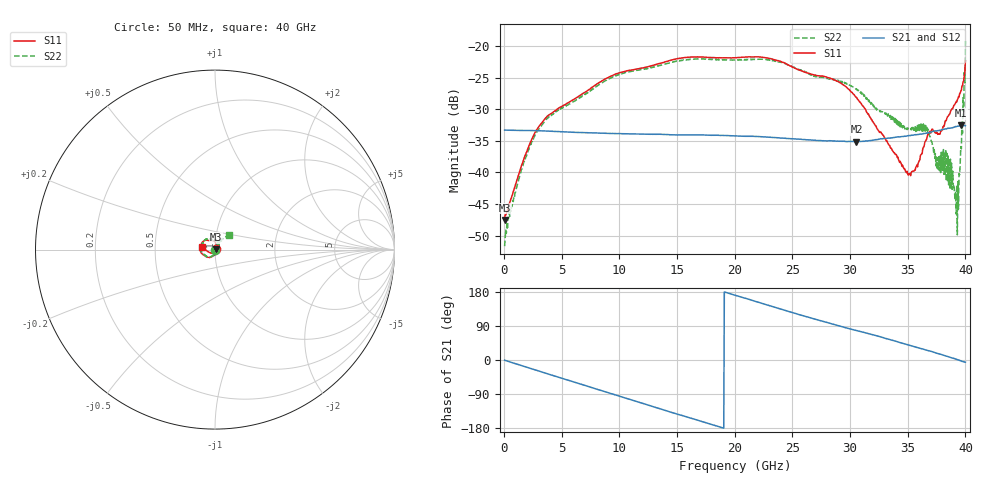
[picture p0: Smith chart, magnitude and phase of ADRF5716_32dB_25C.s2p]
! Device: ADRF5716
! Description: 30GHz 2-Bit Digital Attenuator
! Frequency: 100 MHz – 30 GHz
! Ports:
! ATTIN  = Port 1
! ATTOUT = Port 2
! State: 32 dB Attenuation selected
! Supply Voltage:
! VDD  =  +3.30 Volts
! VSS  =  -3.30 Volts
! Control Voltages:
! D5 = 0V, D6 = 3.3V
! Temperature = +25 C
! Data: Data was collected using a calibrated network analyzer.
!  The reference plane is the package pins of ADRF5716 switch.
! Note: Analog Devices supplies this data as a sample of measured data for this product.
!  Your particular data for this product may vary.
!  Analog Devices reserves the right to change this data at anytime
# HZ S DB R 50
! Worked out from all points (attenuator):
!   800 points, 50 MHz to 40 GHz, reference 50 ohm
!   highest |S21| = -32.55 dB at 39.65 GHz (marker M1); lowest = -35.1 dB at 30.55 GHz (marker M2)
!   lowest |S11| = -47.5 dB at 50 MHz (marker M3), VSWR 1.01, Z = 50.4 + j0.0926 ohm
!   |S11| at or under -10 dB: start of sweep to end of sweep
!   |S22| runs from -51.7 to -19.1 dB; largest |S21 - S12| = 0
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5e7  -47.50 12.6  -33.30 -0.5  -33.30 -0.5  -51.67 -0.2
1.5e9  -38.98 -29.0  -33.35 -14.5  -33.35 -14.5  -39.57 -30.7
2.7e9  -33.63 -60.4  -33.38 -26.0  -33.38 -26.0  -33.97 -62.3
3.95e9  -30.82 -86.3  -33.47 -38.1  -33.47 -38.1  -31.08 -88.8
6.75e9  -27.60 -112.2  -33.68 -64.6  -33.68 -64.6  -28.00 -114.7
9.65e9  -24.44 -134.2  -33.84 -92.1  -33.84 -92.1  -24.68 -136.6
1.34e10  -22.78 -157.7  -33.95 -127.6  -33.95 -127.6  -23.09 -161.7
2.005e10  -21.83 163.7  -34.22 170.7  -34.22 170.7  -22.18 156.7
2.34e10  -22.14 140.9  -34.46 139.9  -34.46 139.9  -22.26 133.1
2.67e10  -24.48 123.1  -34.86 110.1  -34.86 110.1  -24.71 108.8
2.9e10  -25.66 104.5  -35.04 90.5  -35.04 90.5  -25.44 91.2
3.055e10  -28.13 86.4  -35.12 77.9  -35.12 77.9  -26.75 70.1
3.335e10  -35.60 60.8  -34.57 54.7  -34.57 54.7  -31.15 36.8
3.525e10  -40.51 5.1  -34.14 38.1  -34.14 38.1  -32.95 1.7
3.585e10  -39.11 -33.4  -34.02 32.7  -34.02 32.7  -32.57 -11.1
3.665e10  -34.68 -80.2  -33.77 25.9  -33.77 25.9  -32.86 -38.7
3.755e10  -33.71 -123.7  -33.42 17.7  -33.42 17.7  -39.53 -54.1
3.86e10  -30.81 -139.0  -32.99 7.6  -32.99 7.6  -37.80 -76.8
3.92e10  -28.78 -156.6  -32.77 1.9  -32.77 1.9  -46.58 -58.7
3.94e10  -28.03 -162.3  -32.67 -0.0  -32.67 -0.0  -45.79 33.2
3.965e10  -26.99 -169.8  -32.55 -2.8  -32.55 -2.8  -36.27 114.6
4e10  -22.35 170.2  -32.61 -5.7  -32.61 -5.7  -19.11 46.9
